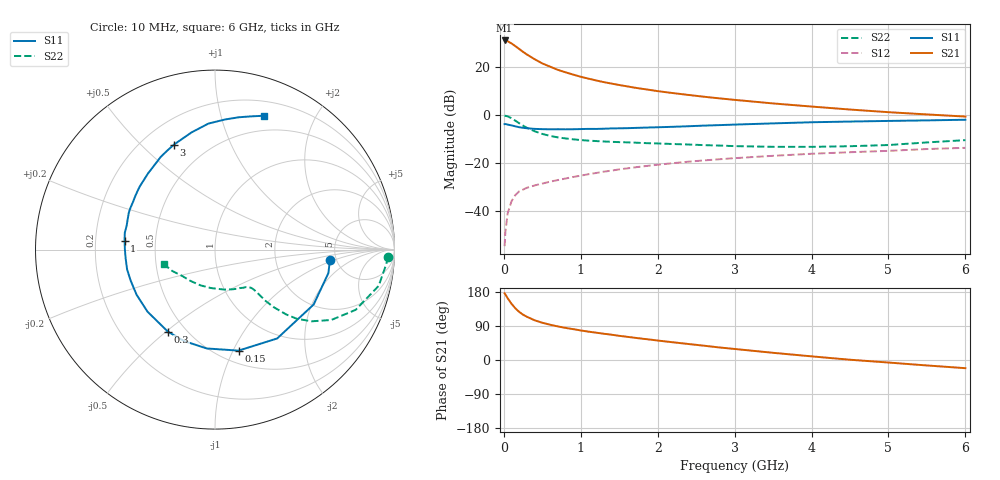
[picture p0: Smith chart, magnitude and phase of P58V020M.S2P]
! SIEMENS Small Signal Semiconductors
! BFP183
! Si NPN RF Bipolar Junction Transistor in SOT143
! VCE = 8 V  IC = 20 mA
! Common Emitter S-Parameters:  March  1996
# GHz  S  MA  R  50
!  f  S11  S21  S12  S22
! GHz  MAG  ANG  MAG  ANG  MAG  ANG  MAG  ANG
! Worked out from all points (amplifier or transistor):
!   36 points, 10 MHz to 6 GHz, reference 50 ohm
!   highest |S21| = 31.2 dB at 10 MHz (marker M1)
!   |S21| within 3 dB of that: start of sweep to 176.2 MHz
!   unconditionally stable (mu >= 1): 946.9 MHz to 5.786 GHz
!   at 250 MHz: K = 0.44, MSG = 28.8 dB, |S12| = -31.2 dB
!   at 1.4 GHz: K = 1.10, MAG = 16.3 dB, |S12| = -23.3 dB
!   at 6 GHz: K = 0.98, MSG = 6.5 dB, |S12| = -13.8 dB
!   S11 on the Smith chart (normalised r, x): 10 MHz: 4.40, -0.91; 150 MHz: 0.62, -1.05; 300 MHz: 0.40, -0.51; 1 GHz: 0.33, +0.04; 3 GHz: 0.33, +0.63; 6 GHz: 0.34, +1.37
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0.01  0.6429 -5.4  36.13 176.0  0.0018 86.6  0.966 -2.4
0.02  0.6452 -11.7  35.8 173.0  0.0036 86.2  0.9572 -5.0
0.05  0.6291 -29.1  34.8 162.9  0.0088 78.5  0.934 -12.5
0.1  0.6043 -55.0  31.28 148.3  0.0157 67.8  0.8525 -23.2
0.15  0.5779 -76.9  27.46 136.3  0.0212 59.4  0.757 -31.2
0.2  0.5527 -94.8  23.98 126.9  0.0252 54.3  0.6702 -36.6
0.25  0.5379 -108.6  20.82 119.5  0.0275 51.1  0.597 -40.2
0.3  0.5272 -119.8  18.37 114.1  0.03 49.5  0.5377 -42.3
0.4  0.511 -137.4  14.63 104.8  0.0335 47.8  0.4558 -44.5
0.5  0.5041 -150.1  11.97 98.3  0.0367 47.7  0.4012 -45.4
0.6  0.5006 -159.7  10.25 93.1  0.0401 47.9  0.365 -45.5
0.7  0.5021 -167.3  8.8 88.7  0.0434 48.8  0.3399 -45.6
0.8  0.5002 -174.3  7.812 84.8  0.0467 49.6  0.3227 -45.7
1  0.5062 174.3  6.284 78.0  0.0537 50.7  0.2984 -46.3
1.1  0.5112 169.5  5.746 74.8  0.0576 50.7  0.2902 -46.9
1.5  0.5254 153.9  4.227 63.8  0.0727 50.5  0.2698 -50.8
2.2  0.5652 131.3  2.863 46.7  0.0981 46.6  0.2465 -62.8
3  0.6283 111.3  2.067 29.1  0.1248 40.2  0.2228 -81.9
3.5  0.6659 101.3  1.741 19.0  0.1397 35.8  0.2154 -96.2
4.5  0.7275 85.5  1.297 0.7  0.1661 27.0  0.2218 -128.3
5.5  0.7693 74.8  1.025 -14.4  0.1936 19.5  0.2662 -153.4
6  0.7935 70.0  0.925 -21.6  0.2052 15.1  0.2973 -164.4
